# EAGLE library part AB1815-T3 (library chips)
Ultra-low current RTC. 55nA quiescent @ 3V. 1.5-3.6V input.
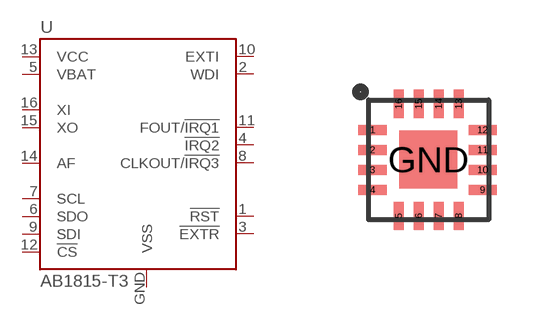
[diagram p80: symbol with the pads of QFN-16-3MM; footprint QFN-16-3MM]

Designator prefix U

## AB1815-T3 (DIGIKEY: 535-11936-1-ND; MANUFACTURER: Abracon; MPN: AB1815-T3)  [QFN-16-3MM]
1  !RST
2  WDI
3  !EXTR
4  !IRQ2
5  VBAT
6  SDO
7  SCL
8  CLKOUT/!IRQ3
9  SDI
10  EXTI
11  FOUT/!IRQ1
12  !CS
13  VCC
14  AF
15  XO
16  XI
GND  VSS

## Footprint QFN-16-3MM (pad centres in mm)
smd 0.7 x 0.25: 1 -1.4,0.75; 2 -1.4,0.25; 3 -1.4,-0.25; 4 -1.4,-0.75; 9 1.35,-0.75; 10 1.35,-0.25; 11 1.35,0.25; 12 1.35,0.75
smd 0.25 x 0.7: 5 -0.75,-1.4; 6 -0.25,-1.4; 7 0.25,-1.4; 8 0.75,-1.4; 13 0.75,1.4; 14 0.25,1.4; 15 -0.25,1.4; 16 -0.75,1.4
smd 1.45 x 1.45: GND 0,0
